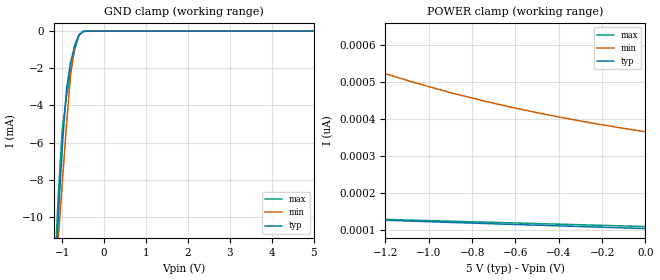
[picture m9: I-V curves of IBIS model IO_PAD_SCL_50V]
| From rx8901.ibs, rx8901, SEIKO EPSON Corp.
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[Model]   IO_PAD_SCL_50V
Model_type Input
Polarity Non-Inverting
Vinh=3.50
Vinl=1.50
C_comp   2.5p   2.0p   3.0p
[Temperature Range] 25   105   -40
[Voltage Range]   5.00   4.50   5.50
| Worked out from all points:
|   GND clamp passes 1 mA (typ) near -0.73 V on its own axis
[GND Clamp]
-5V       -174.9mA   -140.4mA   -216.2mA
-1.2V     -14.35mA   -14.54mA   -14.15mA
-1.1V     -10.3mA    -11.38mA   -9.07mA
-1V       -6.302mA   -8.237mA   -5.327mA
-900mV    -3.193mA   -5.119mA   -3.551mA
-800mV    -1.656mA   -2.372mA   -2.158mA
-700mV    -763.9uA   -783.7uA   -983.1uA
-600mV    -207.7uA   -205.2uA   -228.8uA
-500mV    -21.87uA   -34.9uA    -13.49uA
-300mV    -47.01nA   -341.4nA   -3.545nA
5V        104.1pA    416.4pA    99.77pA
[POWER Clamp]
-5V       237.4pA    2.814nA    194.9pA
-4.4V     212.3pA    2.152nA    181.1pA
-3.6V     185pA      1.486nA    167.4pA
-2.7V     159.9pA    976.3pA    152.8pA
-1.7V     136.7pA    631.2pA    136.7pA
-1.5V     132.5pA    583.2pA    133.5pA
-1.3V     128.5pA    540.9pA    130.3pA
-1.1V     124.5pA    503.5pA    127.1pA
-900mV    120.6pA    470.7pA    123.9pA
-500mV    113.1pA    416.4pA    117.5pA
-300mV    109.5pA    394pA      114.3pA
0V        104.1pA    365pA      109.5pA
